(* Logix 5000 AddOnInstructionDefinition export Banner_DXMR_IOLM_Param_v4; software revision 33.03 *)

TYPE Banner_IOL_Port_v4 :   // UDT that has all of the data items necessary to communicate with a specific Port on a IO-Link Master
STRUCT
   Port_Controlled : INT;   // Each bit represents a port on an IO-Link Master. Set to 1 to tell AOI to control that port.
   Port_Activate : INT;   // Each bit represents a port on an IO-Link Master. When ON that port will process any commands in queue.
   Port_Read : INT;   // Each bit represents a port on an IO-Link Master. Used to determine when device AOI has requested a Read command.
   Port_Write : INT;   // Each bit represents a port on an IO-Link Master. Used to determine when device AOI has requested a Write command.
   Port_RW_Complete : INT;   // Each bit represents a port on an IO-Link Master. Tells device AOI that Read or Write request has been completed.
   Port_Device_Read : INT;
   Data_Transfer : SINT[190];   // Array to transfer data from IO-Master to device AOIs.
END_STRUCT
END_TYPE

TYPE Banner_IOLM_EL_v4 :   // Error Log for Messages to IOLM.
STRUCT
   RW : SINT;   // 0 = Read, 1 = Write.
   Port : SINT;   // Port number that generated error.
   Index : INT;   // IO-Link Index for generated error.
END_STRUCT
END_TYPE

TYPE Banner_IOLM_v4 :   // UDT to control IO-Link Masters.
STRUCT
   Message_Source_Data : SINT[190];
   Message_Destination_Data : SINT[190];
   Error_Log : Banner_IOLM_EL_v4[10];
   Error_Write_Retry : BOOL;
   Num_Error_MSGS : DINT;
   IO_Link_Master_Busy : BOOL;   // 0 = While waiting for a command, 1 = Processing command
   AOI_Reset : BOOL;
   Port_Data : Banner_IOL_Port_v4;   // All of the necessary data to work with the various ports of the IO-Link Master.
   Halt_Operation : BOOL;   // When parameter is 1 the AOI is halted as next available time frame.
   AOI_Halted : BOOL;   // AOI is in standby mode until Halt Operation tag is set back to 0.
END_STRUCT
END_TYPE

ADD_ON_INSTRUCTION Banner_DXMR_IOLM_Param_v4   (* revision 4.4, vendor Banner Engineering *)
// AOI that controls a Banner IO-Link Master with Banner devices for parameter data operations.
// Revision note:
// Timer Presets have added code.
VAR_IN_OUT
   IOLM : Banner_IOLM_v4; {required}
END_VAR
VAR
   Lock : DINT; {access None}
   Byte_Length : SINT; {access None}
   Current_Port : INT; {access None}   // Current port to communicate with via the IO-Link Master.
   Timer1 : TIMER := (PRE := 500); {access None}
   Error_Index : DINT; {access None}
   Timer2 : TIMER := (PRE := 5000); {access None}
   Temp_Index : INT; {access None}
   ErrCount : DINT; {access None}
   Timer4 : TIMER := (PRE := 2000); {access None}
   Timer5 : TIMER := (PRE := 2000); {access None}
   Timer3 : TIMER := (PRE := 2000); {access None}
   Timer6 : TIMER := (PRE := 3000); {access None}
   Timer7 : TIMER := (PRE := 3000); {access None}
   Timer8 : TIMER := (PRE := 3000); {access None}
END_VAR

ROUTINE Logic   (* ladder *)
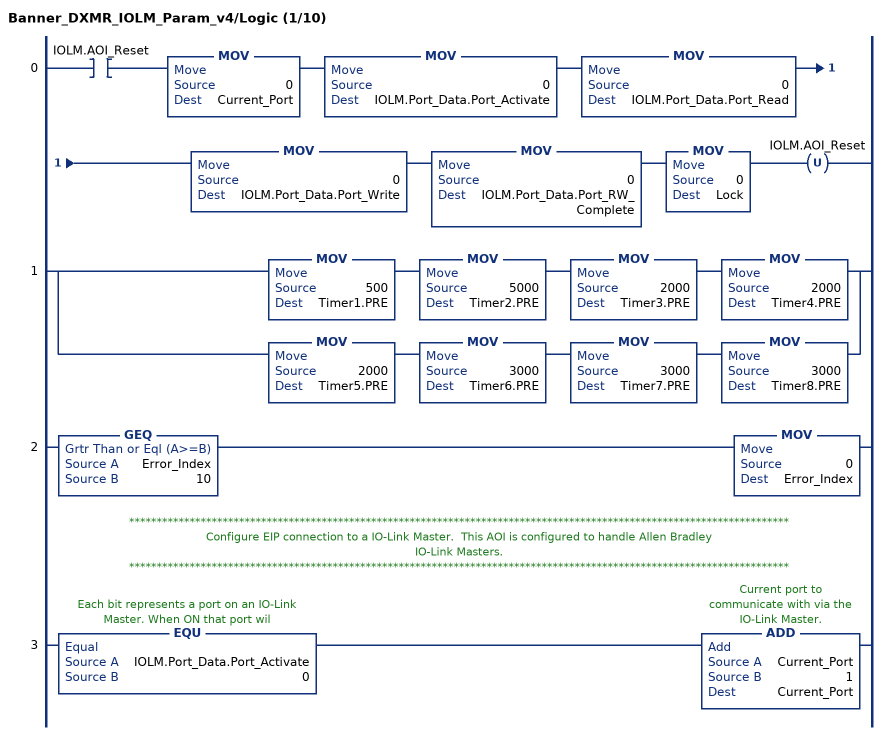
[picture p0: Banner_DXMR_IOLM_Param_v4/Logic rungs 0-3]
   0: XIC(IOLM.AOI_Reset)MOV(0,Current_Port)MOV(0,IOLM.Port_Data.Port_Activate)MOV(0,IOLM.Port_Data.Port_Read)MOV(0,IOLM.Port_Data.Port_Write)MOV(0,IOLM.Port_Data.Port_RW_Complete)MOV(0,Lock)OTU(IOLM.AOI_Reset);
   1: [MOV(500,Timer1.PRE) MOV(5000,Timer2.PRE) MOV(2000,Timer3.PRE) MOV(2000,Timer4.PRE) ,MOV(2000,Timer5.PRE) MOV(3000,Timer6.PRE) MOV(3000,Timer7.PRE) MOV(3000,Timer8.PRE) ];
   2: GEQ(Error_Index,10)MOV(0,Error_Index);
   // ************************************************************************************************************************
   // Configure EIP connection to a IO-Link Master.  This AOI is configured to handle Allen Bradley
   // IO-Link Masters.
   // ************************************************************************************************************************
   3: EQU(IOLM.Port_Data.Port_Activate,0)ADD(Current_Port,1,Current_Port);
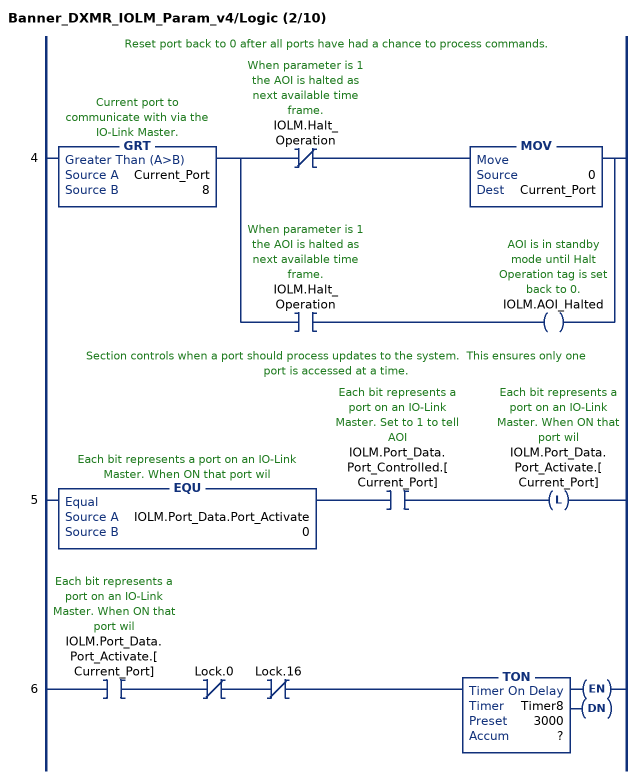
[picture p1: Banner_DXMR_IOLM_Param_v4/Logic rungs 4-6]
   // Reset port back to 0 after all ports have had a chance to process commands.
   4: GRT(Current_Port,8)[XIO(IOLM.Halt_Operation) MOV(0,Current_Port) ,XIC(IOLM.Halt_Operation) OTE(IOLM.AOI_Halted) ];
   // Section controls when a port should process updates to the system.  This ensures only one port is accessed at a time.
   5: EQU(IOLM.Port_Data.Port_Activate,0)XIC(IOLM.Port_Data.Port_Controlled.[Current_Port])OTL(IOLM.Port_Data.Port_Activate.[Current_Port]);
   6: XIC(IOLM.Port_Data.Port_Activate.[Current_Port])XIO(Lock.0)XIO(Lock.16)TON(Timer8,?,?);
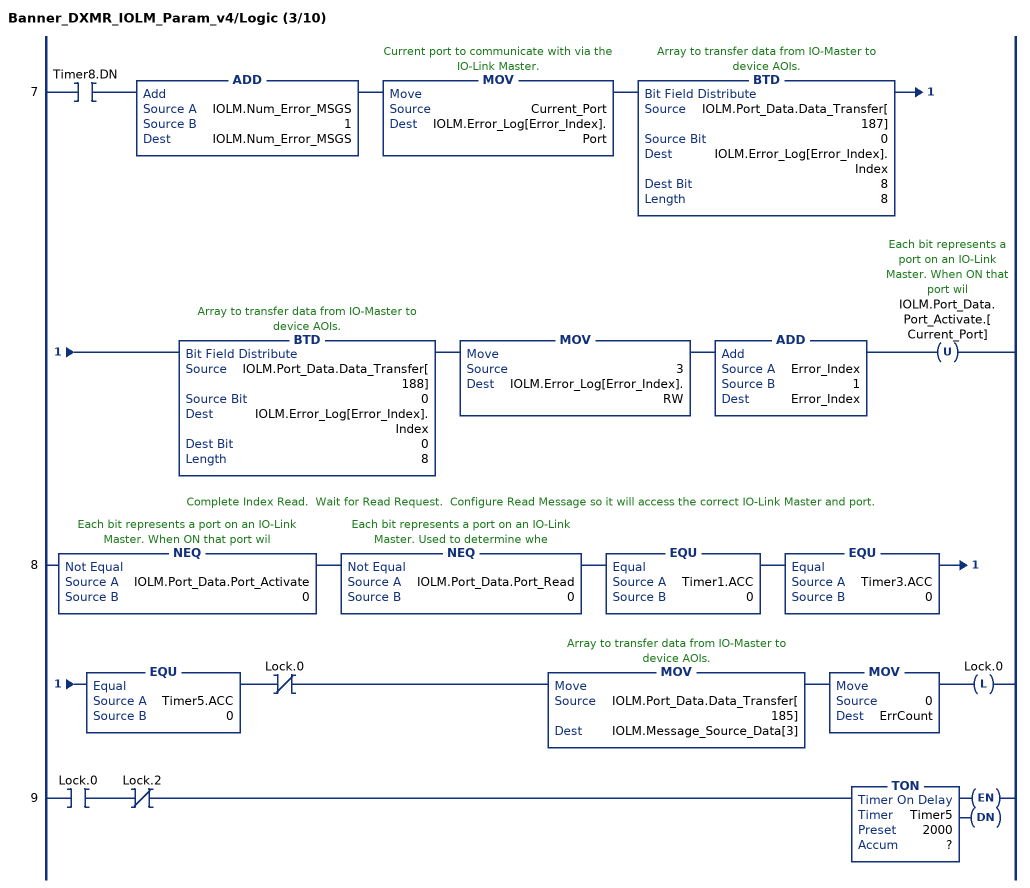
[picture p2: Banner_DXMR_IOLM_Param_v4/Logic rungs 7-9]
   7: XIC(Timer8.DN)ADD(IOLM.Num_Error_MSGS,1,IOLM.Num_Error_MSGS)MOV(Current_Port,IOLM.Error_Log[Error_Index].Port)BTD(IOLM.Port_Data.Data_Transfer[187],0,IOLM.Error_Log[Error_Index].Index,8,8)BTD(IOLM.Port_Data.Data_Transfer[188],0,IOLM.Error_Log[Error_Index].Index,0,8)MOV(3,IOLM.Error_Log[Error_Index].RW)ADD(Error_Index,1,Error_Index)OTU(IOLM.Port_Data.Port_Activate.[Current_Port]);
   // Complete Index Read.  Wait for Read Request.  Configure Read Message so it will access the correct IO-Link Master and port.
   8: NEQ(IOLM.Port_Data.Port_Activate,0)NEQ(IOLM.Port_Data.Port_Read,0)EQU(Timer1.ACC,0)EQU(Timer3.ACC,0)EQU(Timer5.ACC,0)XIO(Lock.0)MOV(IOLM.Port_Data.Data_Transfer[185],IOLM.Message_Source_Data[3])MOV(0,ErrCount)OTL(Lock.0);
   9: XIC(Lock.0)XIO(Lock.2)TON(Timer5,?,?);
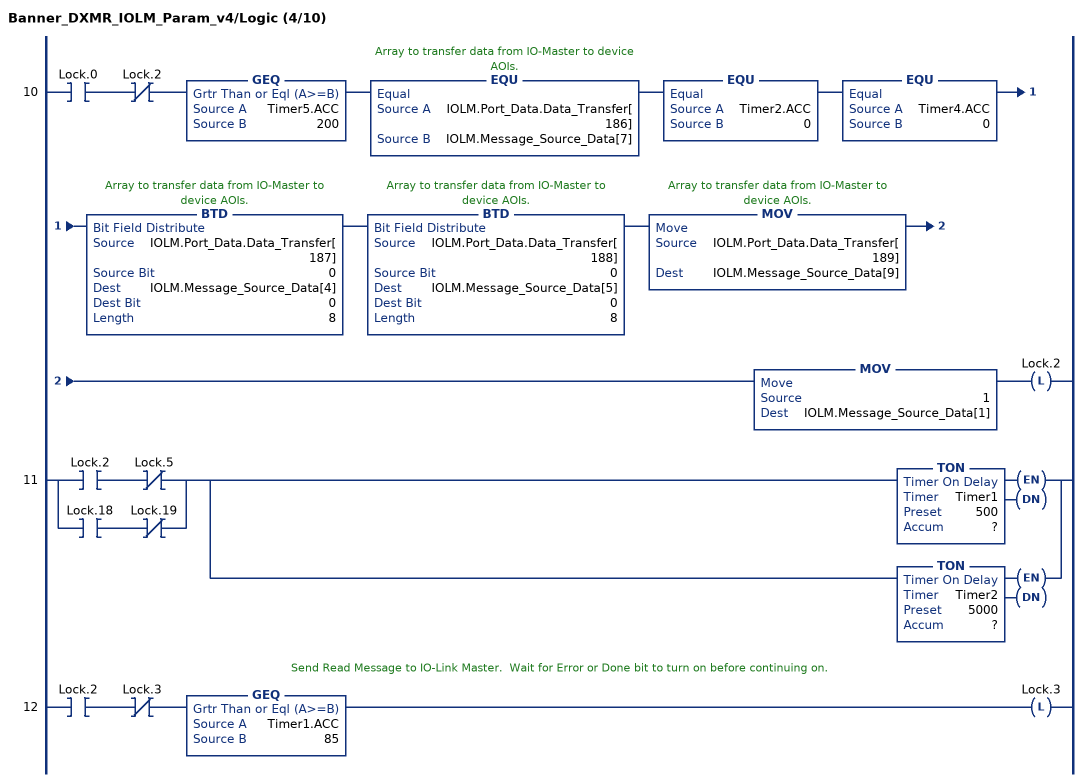
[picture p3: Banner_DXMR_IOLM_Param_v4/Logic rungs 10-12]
   10: XIC(Lock.0)XIO(Lock.2)GEQ(Timer5.ACC,200)EQU(IOLM.Port_Data.Data_Transfer[186],IOLM.Message_Source_Data[7])EQU(Timer2.ACC,0)EQU(Timer4.ACC,0)BTD(IOLM.Port_Data.Data_Transfer[187],0,IOLM.Message_Source_Data[4],0,8)BTD(IOLM.Port_Data.Data_Transfer[188],0,IOLM.Message_Source_Data[5],0,8)MOV(IOLM.Port_Data.Data_Transfer[189],IOLM.Message_Source_Data[9])MOV(1,IOLM.Message_Source_Data[1])OTL(Lock.2);
   11: [XIC(Lock.2) XIO(Lock.5) ,XIC(Lock.18) XIO(Lock.19) ][TON(Timer1,?,?) ,TON(Timer2,?,?) ];
   // Send Read Message to IO-Link Master.  Wait for Error or Done bit to turn on before continuing on.
   12: XIC(Lock.2)XIO(Lock.3)GEQ(Timer1.ACC,85)OTL(Lock.3);
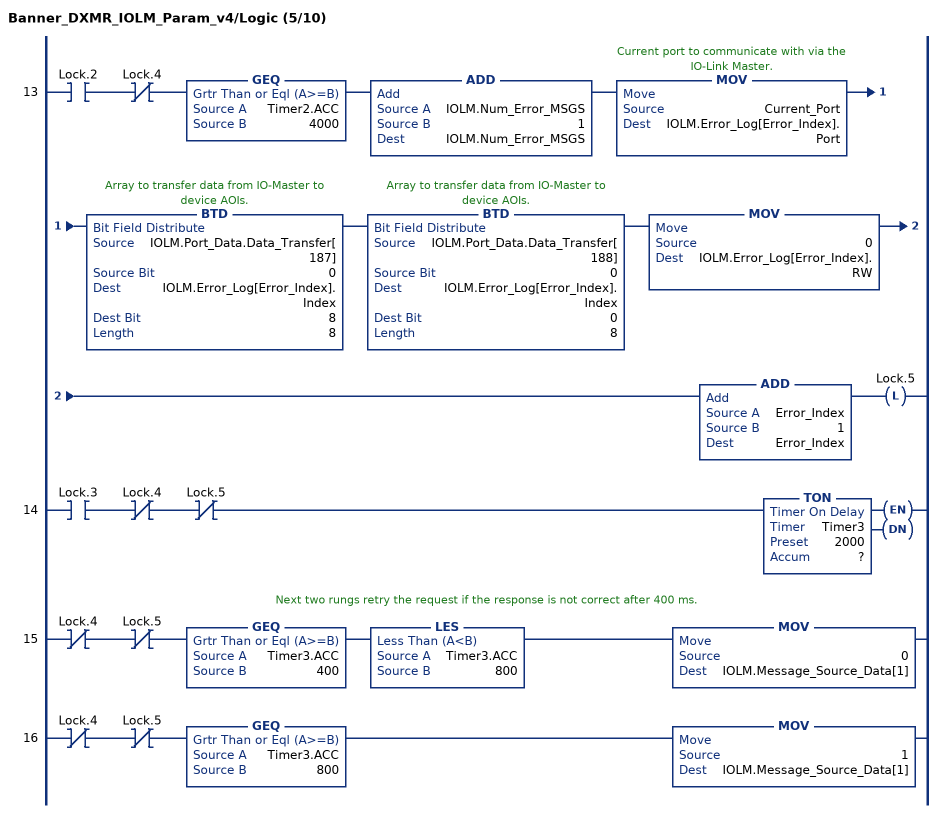
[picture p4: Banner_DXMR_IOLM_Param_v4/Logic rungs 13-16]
   13: XIC(Lock.2)XIO(Lock.4)GEQ(Timer2.ACC,4000)ADD(IOLM.Num_Error_MSGS,1,IOLM.Num_Error_MSGS)MOV(Current_Port,IOLM.Error_Log[Error_Index].Port)BTD(IOLM.Port_Data.Data_Transfer[187],0,IOLM.Error_Log[Error_Index].Index,8,8)BTD(IOLM.Port_Data.Data_Transfer[188],0,IOLM.Error_Log[Error_Index].Index,0,8)MOV(0,IOLM.Error_Log[Error_Index].RW)ADD(Error_Index,1,Error_Index)OTL(Lock.5);
   14: XIC(Lock.3)XIO(Lock.4)XIO(Lock.5)TON(Timer3,?,?);
   // Next two rungs retry the request if the response is not correct after 400 ms.
   15: XIO(Lock.4)XIO(Lock.5)GEQ(Timer3.ACC,400)LES(Timer3.ACC,800)MOV(0,IOLM.Message_Source_Data[1]);
   16: XIO(Lock.4)XIO(Lock.5)GEQ(Timer3.ACC,800)MOV(1,IOLM.Message_Source_Data[1]);
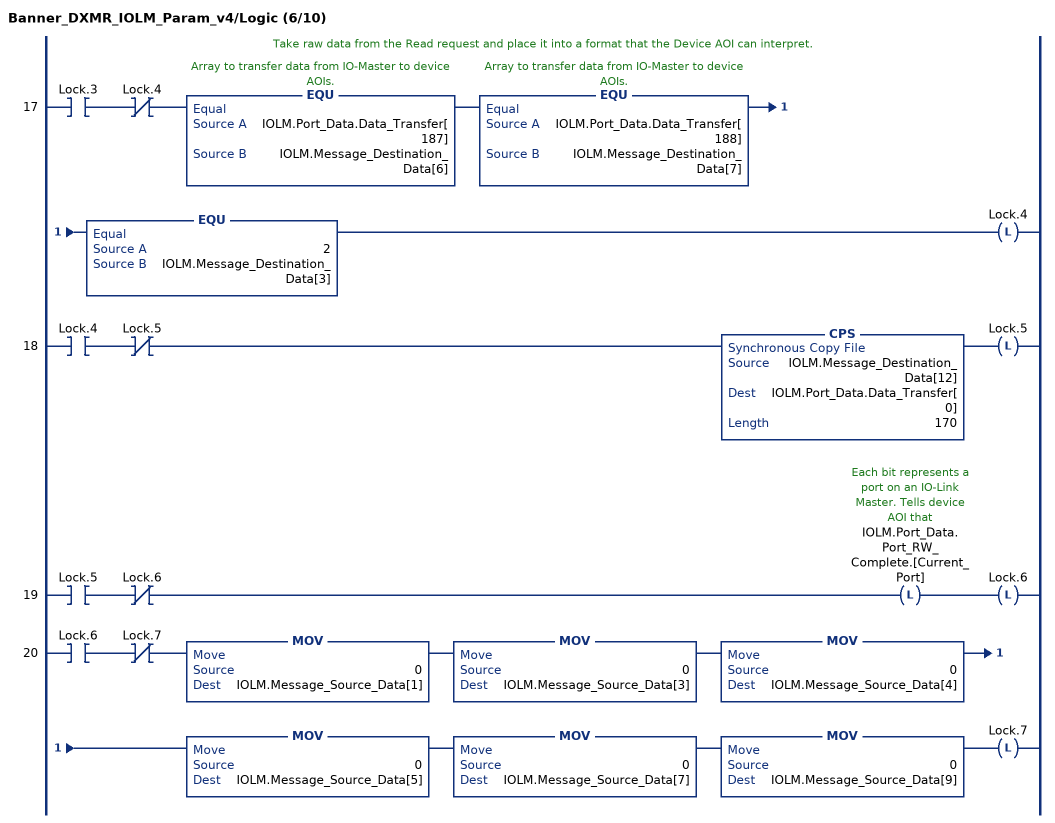
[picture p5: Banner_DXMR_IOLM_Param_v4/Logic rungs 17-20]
   // Take raw data from the Read request and place it into a format that the Device AOI can interpret.
   17: XIC(Lock.3)XIO(Lock.4)EQU(IOLM.Port_Data.Data_Transfer[187],IOLM.Message_Destination_Data[6])EQU(IOLM.Port_Data.Data_Transfer[188],IOLM.Message_Destination_Data[7])EQU(2,IOLM.Message_Destination_Data[3])OTL(Lock.4);
   18: XIC(Lock.4)XIO(Lock.5)CPS(IOLM.Message_Destination_Data[12],IOLM.Port_Data.Data_Transfer[0],170)OTL(Lock.5);
   19: XIC(Lock.5)XIO(Lock.6)OTL(IOLM.Port_Data.Port_RW_Complete.[Current_Port])OTL(Lock.6);
   20: XIC(Lock.6)XIO(Lock.7)MOV(0,IOLM.Message_Source_Data[1])MOV(0,IOLM.Message_Source_Data[3])MOV(0,IOLM.Message_Source_Data[4])MOV(0,IOLM.Message_Source_Data[5])MOV(0,IOLM.Message_Source_Data[7])MOV(0,IOLM.Message_Source_Data[9])OTL(Lock.7);
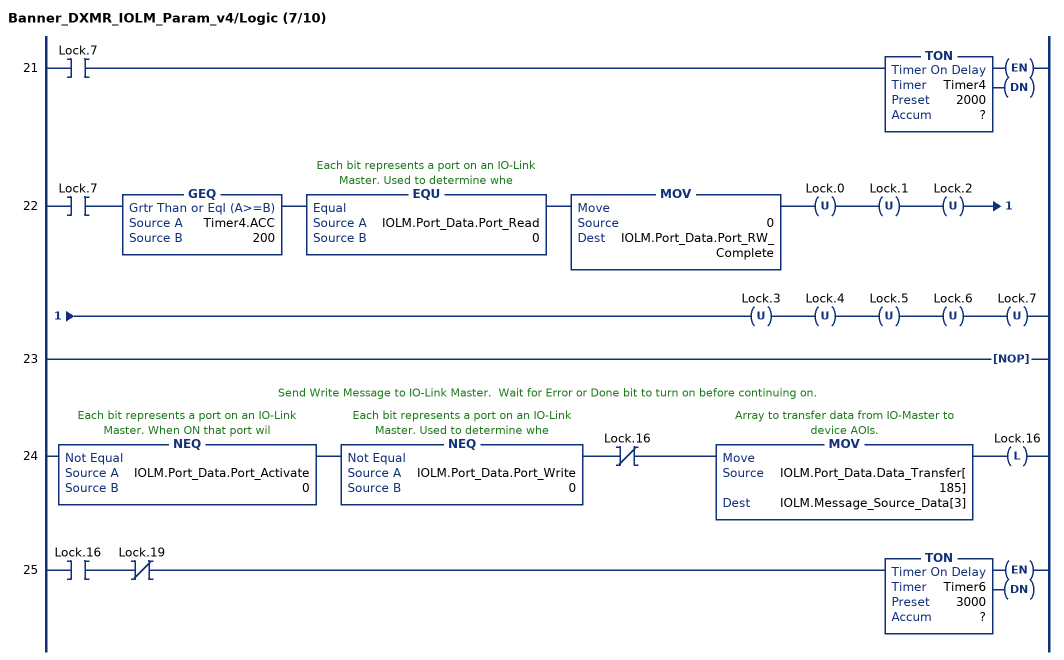
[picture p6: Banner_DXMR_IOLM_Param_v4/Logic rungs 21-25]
   21: XIC(Lock.7)TON(Timer4,?,?);
   22: XIC(Lock.7)GEQ(Timer4.ACC,200)EQU(IOLM.Port_Data.Port_Read,0)MOV(0,IOLM.Port_Data.Port_RW_Complete)OTU(Lock.0)OTU(Lock.1)OTU(Lock.2)OTU(Lock.3)OTU(Lock.4)OTU(Lock.5)OTU(Lock.6)OTU(Lock.7);
   23: NOP();
   // Send Write Message to IO-Link Master.  Wait for Error or Done bit to turn on before continuing on.
   24: NEQ(IOLM.Port_Data.Port_Activate,0)NEQ(IOLM.Port_Data.Port_Write,0)XIO(Lock.16)MOV(IOLM.Port_Data.Data_Transfer[185],IOLM.Message_Source_Data[3])OTL(Lock.16);
   25: XIC(Lock.16)XIO(Lock.19)TON(Timer6,?,?);
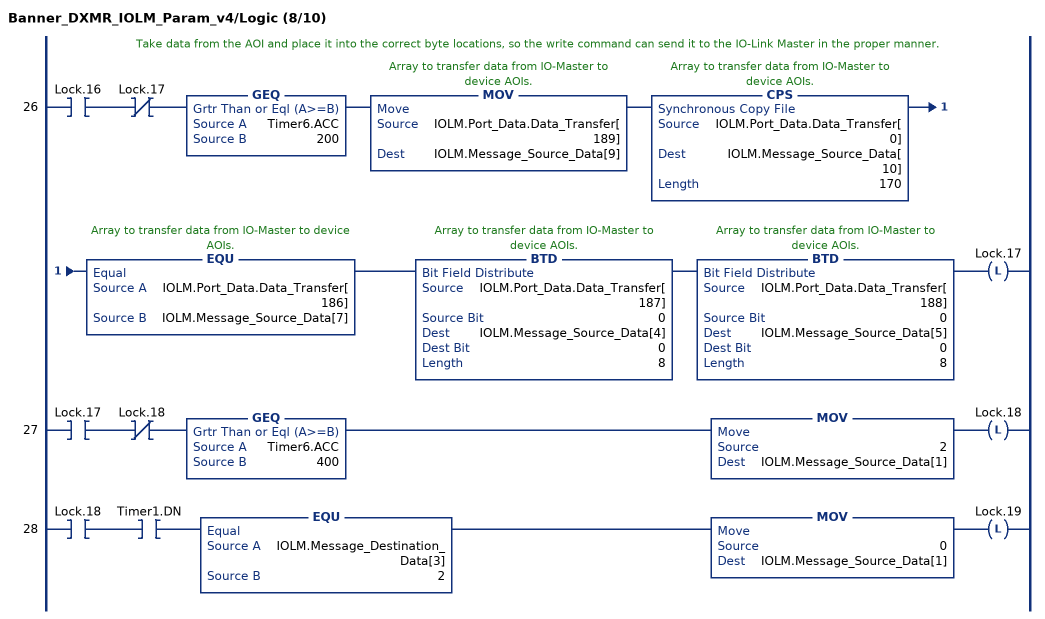
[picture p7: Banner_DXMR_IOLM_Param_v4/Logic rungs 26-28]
   // Take data from the AOI and place it into the correct byte locations, so the write command can send it to the IO-Link Master in the proper manner.
   26: XIC(Lock.16)XIO(Lock.17)GEQ(Timer6.ACC,200)MOV(IOLM.Port_Data.Data_Transfer[189],IOLM.Message_Source_Data[9])CPS(IOLM.Port_Data.Data_Transfer[0],IOLM.Message_Source_Data[10],170)EQU(IOLM.Port_Data.Data_Transfer[186],IOLM.Message_Source_Data[7])BTD(IOLM.Port_Data.Data_Transfer[187],0,IOLM.Message_Source_Data[4],0,8)BTD(IOLM.Port_Data.Data_Transfer[188],0,IOLM.Message_Source_Data[5],0,8)OTL(Lock.17);
   27: XIC(Lock.17)XIO(Lock.18)GEQ(Timer6.ACC,400)MOV(2,IOLM.Message_Source_Data[1])OTL(Lock.18);
   28: XIC(Lock.18)XIC(Timer1.DN)EQU(IOLM.Message_Destination_Data[3],2)MOV(0,IOLM.Message_Source_Data[1])OTL(Lock.19);
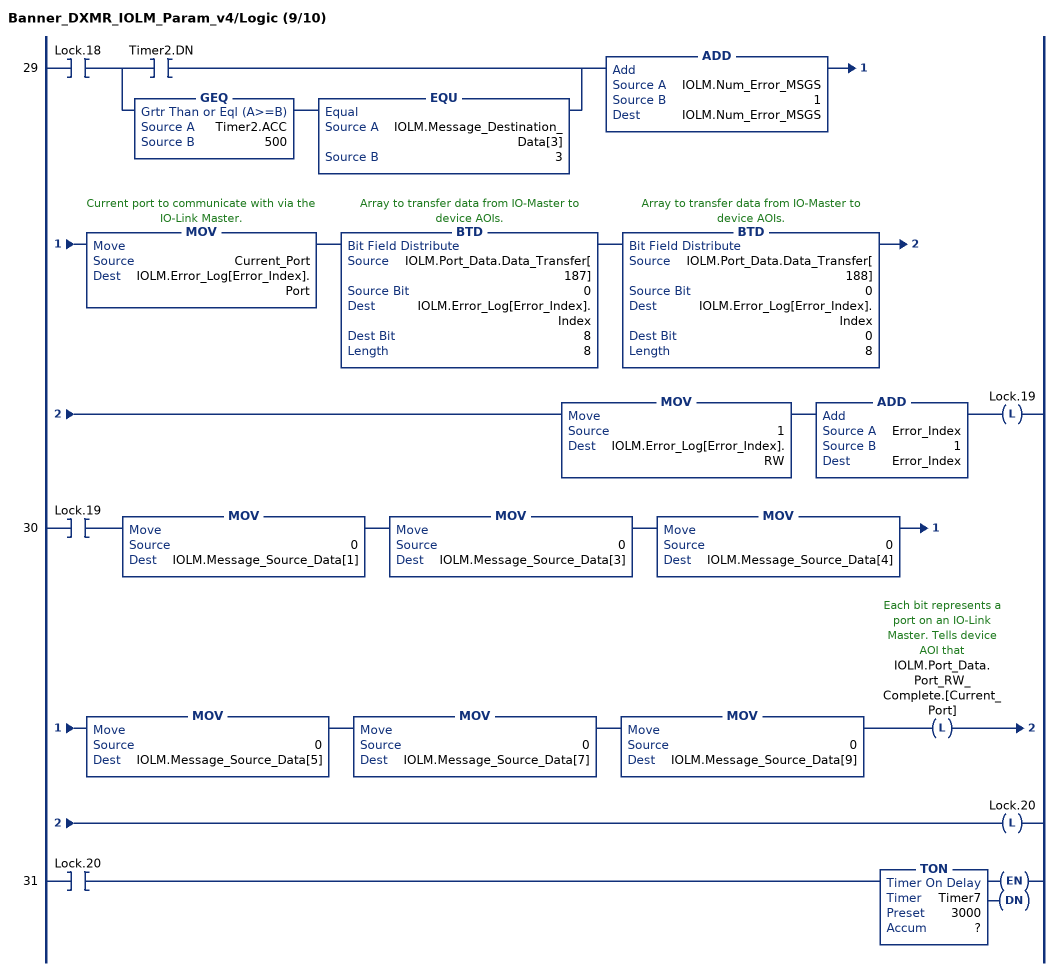
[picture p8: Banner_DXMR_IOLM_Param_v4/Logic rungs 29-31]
   29: XIC(Lock.18)[XIC(Timer2.DN) ,GEQ(Timer2.ACC,500) EQU(IOLM.Message_Destination_Data[3],3) ]ADD(IOLM.Num_Error_MSGS,1,IOLM.Num_Error_MSGS)MOV(Current_Port,IOLM.Error_Log[Error_Index].Port)BTD(IOLM.Port_Data.Data_Transfer[187],0,IOLM.Error_Log[Error_Index].Index,8,8)BTD(IOLM.Port_Data.Data_Transfer[188],0,IOLM.Error_Log[Error_Index].Index,0,8)MOV(1,IOLM.Error_Log[Error_Index].RW)ADD(Error_Index,1,Error_Index)OTL(Lock.19);
   30: XIC(Lock.19)MOV(0,IOLM.Message_Source_Data[1])MOV(0,IOLM.Message_Source_Data[3])MOV(0,IOLM.Message_Source_Data[4])MOV(0,IOLM.Message_Source_Data[5])MOV(0,IOLM.Message_Source_Data[7])MOV(0,IOLM.Message_Source_Data[9])OTL(IOLM.Port_Data.Port_RW_Complete.[Current_Port])OTL(Lock.20);
   31: XIC(Lock.20)TON(Timer7,?,?);
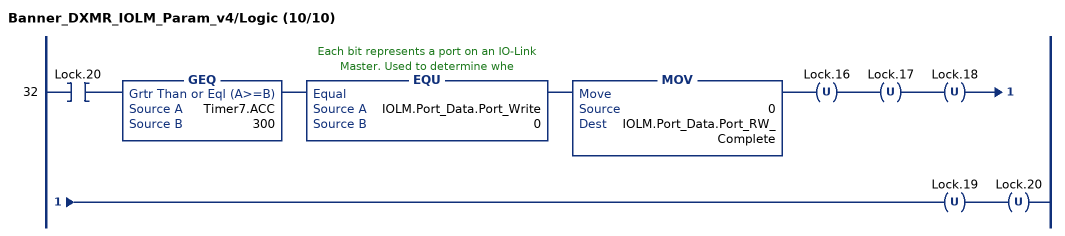
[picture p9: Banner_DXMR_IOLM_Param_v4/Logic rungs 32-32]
   32: XIC(Lock.20)GEQ(Timer7.ACC,300)EQU(IOLM.Port_Data.Port_Write,0)MOV(0,IOLM.Port_Data.Port_RW_Complete)OTU(Lock.16)OTU(Lock.17)OTU(Lock.18)OTU(Lock.19)OTU(Lock.20);
END_ROUTINE
END_ADD_ON_INSTRUCTION
